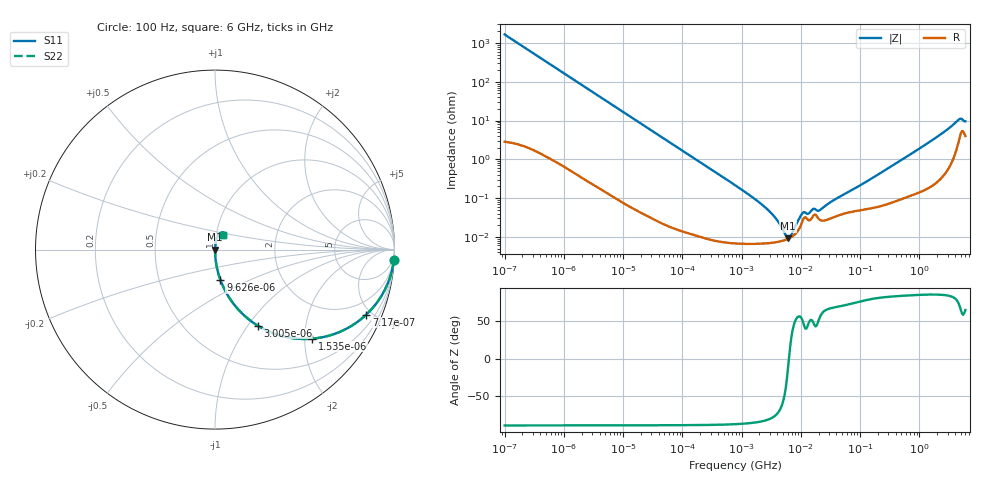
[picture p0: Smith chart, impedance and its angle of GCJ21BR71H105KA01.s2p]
!Murata Part Number: GCJ21BR71H105KA01
!These Parameters are Measured in Series Mode Connection
!Data Generated on Mar 13, 2026
!  o--ll--o
!Port1  Port2
!  o------o
!Operation Temp=25[degC], DC Bias Voltage=0[V]
!Freq. Start=100[Hz] Stop=6[GHz] 401[Steps]
# Hz S RI R 50
!Freq.(Hz) S11(Real) S11(Imag) S21(Real) S21(Imag) S12(Real) S12(Imag) S22(Real) S22(Imag)
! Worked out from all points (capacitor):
!   401 points, 100 Hz to 6 GHz, reference 50 ohm
!   read as one part in series: C = 959 nF near 109 Hz
!   lowest |Z| = 9.14 mohm at 6.075 MHz (marker M1)
!   series resonance near 6.304 MHz, so ESL is about 660 pH
!   S11 on the Smith chart (normalised r, x): 100 Hz: 1, -33; 717 Hz: 1.02, -4.64; 1.535 kHz: 1.01, -2.17; 3.005 kHz: 1.00, -1.11; 9.626 kHz: 1.00, -0.35; 6 GHz: 1.08, +0.17
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100  0.9963 -0.0601  0.00373 0.0601  0.00373 0.0601  0.9963 -0.0601
335  0.9604 -0.1935  0.0396 0.1935  0.0396 0.1935  0.9604 -0.1935
717  0.8425 -0.3624  0.1575 0.3624  0.1575 0.3624  0.8425 -0.3624
1535  0.5412 -0.4963  0.4588 0.4963  0.4588 0.4963  0.5412 -0.4963
2008  0.4089 -0.4896  0.5911 0.4896  0.5911 0.4896  0.4089 -0.4896
3005  0.2371 -0.4232  0.7629 0.4232  0.7629 0.4232  0.2371 -0.4232
5143  0.0967 -0.2935  0.9033 0.2935  0.9033 0.2935  0.0967 -0.2935
9626  0.0301 -0.1687  0.9699 0.1687  0.9699 0.1687  0.0301 -0.1687
40335  0.00198 -0.0416  0.998 0.0416  0.998 0.0416  0.00198 -0.0416
774597  7.22e-05 -0.00216  0.9999 0.00216  0.9999 0.00216  7.22e-05 -0.00216
2837864  6.88e-05 -0.00048  0.9999 0.00048  0.9999 0.00048  6.88e-05 -0.00048
3882480  7.31e-05 -0.000275  0.9999 0.000275  0.9999 0.000275  7.31e-05 -0.000275
5311619  8.22e-05 -9.52e-05  0.9999 9.52e-05  0.9999 9.52e-05  8.22e-05 -9.52e-05
6075234  8.9e-05 -2.06e-05  0.9999 2.06e-05  0.9999 2.06e-05  8.9e-05 -2.06e-05
6948629  9.92e-05 5.57e-05  0.9999 -5.57e-05  0.9999 -5.57e-05  9.92e-05 5.57e-05
1.039699e7  0.000229 0.000311  0.9998 -0.000311  0.9998 -0.000311  0.000229 0.000311
1.555665e7  0.000314 0.00039  0.9997 -0.00039  0.9997 -0.00039  0.000314 0.00039
2.128304e7  0.000271 0.000415  0.9997 -0.000415  0.9997 -0.000415  0.000271 0.000415
3.124326e8  0.00076 0.0061  0.9992 -0.0061  0.9992 -0.0061  0.00076 0.0061
1.873145e9  0.00361 0.0352  0.9964 -0.0352  0.9964 -0.0352  0.00361 0.0352
4.586474e9  0.0362 0.0942  0.9638 -0.0942  0.9638 -0.0942  0.0362 0.0942
6e9  0.045 0.08  0.955 -0.08  0.955 -0.08  0.045 0.08
